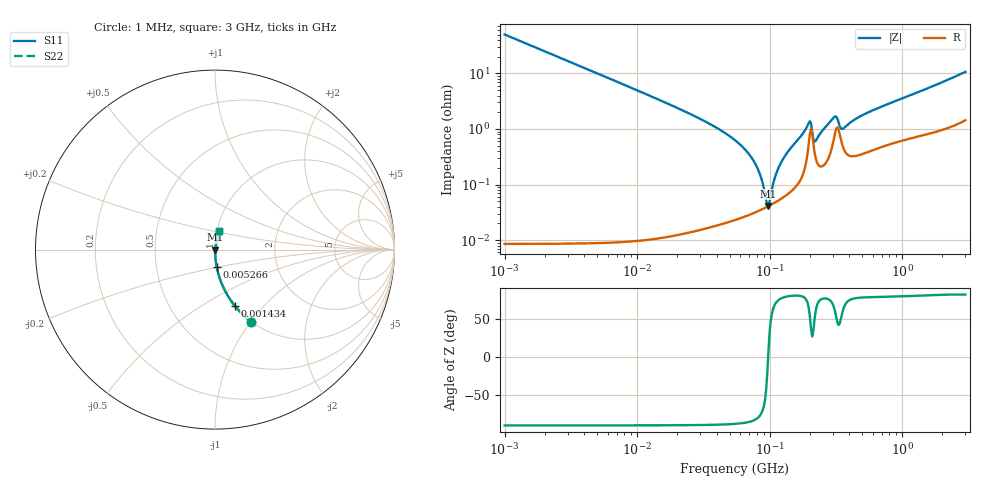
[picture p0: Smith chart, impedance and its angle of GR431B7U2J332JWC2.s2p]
!Murata Part Number: GR431B7U2J332JWC2
!These Parameters are Measured in Series Mode Connection
!Data Generated on Jun 10, 2025
!  o--ll--o
!Port1  Port2
!  o------o
!Operation Temp=25[degC], DC Bias Voltage=0[V]
!Freq. Start=1000[kHz] Stop=3[GHz] 401[Steps]
# Hz S RI R 50
!Freq.(Hz) S11(Real) S11(Imag) S21(Real) S21(Imag) S12(Real) S12(Imag) S22(Real) S22(Imag)
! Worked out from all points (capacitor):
!   401 points, 1 MHz to 3 GHz, reference 50 ohm
!   read as one part in series: C = 3.17 nF near 1.041 MHz
!   lowest |Z| = 41.1 mohm at 97.87 MHz (marker M1)
!   series resonance near 97.43 MHz, so ESL is about 840 pH
!   S11 on the Smith chart (normalised r, x): 1 MHz: 1.00, -1.01; 1.434 MHz: 1.00, -0.70; 5.266 MHz: 1.00, -0.19; 3 GHz: 1.03, +0.21
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1000000  0.2017 -0.4012  0.7983 0.4012  0.7983 0.4012  0.2017 -0.4012
1433740  0.1095 -0.3121  0.8905 0.3121  0.8905 0.3121  0.1095 -0.3121
3823119  0.017 -0.129  0.983 0.129  0.983 0.129  0.017 -0.129
5266264  0.00906 -0.0943  0.9909 0.0943  0.9909 0.0943  0.00906 -0.0943
1.461624e7  0.00124 -0.0336  0.9988 0.0336  0.9988 0.0336  0.00124 -0.0336
3.387922e7  0.000334 -0.013  0.9997 0.013  0.9997 0.013  0.000334 -0.013
5.477226e7  0.00027 -0.00629  0.9997 0.00629  0.9997 0.00629  0.00027 -0.00629
6.690964e7  0.000288 -0.00399  0.9997 0.00399  0.9997 0.00399  0.000288 -0.00399
7.697298e7  0.000318 -0.00247  0.9997 0.00247  0.9997 0.00247  0.000318 -0.00247
8.507507e7  0.000349 -0.00142  0.9997 0.00142  0.9997 0.00142  0.000349 -0.00142
9.402997e7  0.000389 -0.000372  0.9996 0.000372  0.9996 0.000372  0.000389 -0.000372
9.787052e7  0.000409 4.81e-05  0.9996 -4.81e-05  0.9996 -4.81e-05  0.000409 4.81e-05
1.125904e8  0.000494 0.00154  0.9995 -0.00154  0.9995 -0.00154  0.000494 0.00154
1.295243e8  0.00062 0.00313  0.9994 -0.00313  0.9994 -0.00313  0.00062 0.00313
1.971969e8  0.00553 0.0115  0.9945 -0.0115  0.9945 -0.0115  0.00553 0.0115
2.094008e8  0.00816 0.00415  0.9918 -0.00415  0.9918 -0.00415  0.00816 0.00415
2.223601e8  0.00304 0.00528  0.997 -0.00528  0.997 -0.00528  0.00304 0.00528
3.062963e8  0.00708 0.0146  0.9929 -0.0146  0.9929 -0.0146  0.00708 0.0146
3.594878e8  0.00465 0.00901  0.9954 -0.00901  0.9954 -0.00901  0.00465 0.00901
4.853736e8  0.00372 0.0166  0.9963 -0.0166  0.9963 -0.0166  0.00372 0.0166
8.005644e8  0.00604 0.028  0.994 -0.028  0.994 -0.028  0.00604 0.028
3e9  0.0248 0.1017  0.9752 -0.1017  0.9752 -0.1017  0.0248 0.1017
